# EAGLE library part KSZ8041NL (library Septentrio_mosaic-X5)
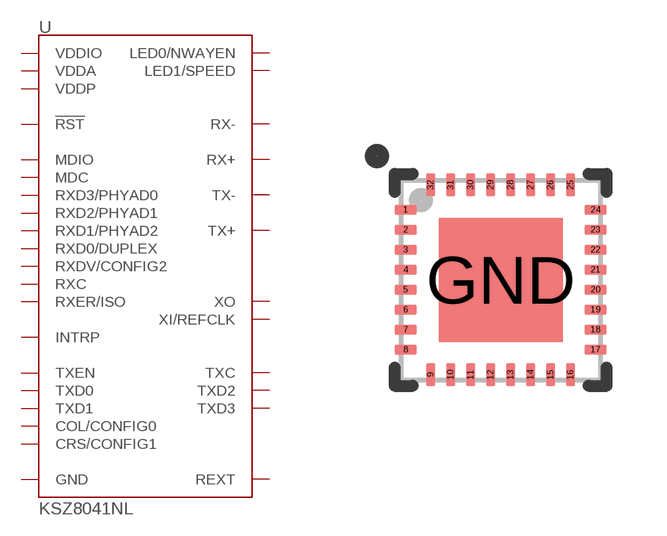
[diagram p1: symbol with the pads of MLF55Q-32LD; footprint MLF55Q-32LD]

Designator prefix -

## KSZ8041NL (PROD_ID: IC-19428; VALUE: KSZ8041NLI)  [MLF55Q-32LD]
1  GND  pwr
2  VDDP
3  VDDA  pwr
4  RX-
5  RX+
6  TX-
7  TX+
8  XO
9  XI/REFCLK
10  REXT
11  MDIO
12  MDC
13  RXD3/PHYAD0
14  RXD2/PHYAD1
15  RXD1/PHYAD2
16  RXD0/DUPLEX
17  VDDIO  pwr
18  RXDV/CONFIG2
19  RXC
20  RXER/ISO
21  INTRP
22  TXC
23  TXEN
24  TXD0
25  TXD1
26  TXD2
27  TXD3
28  COL/CONFIG0
29  CRS/CONFIG1
30  LED0/NWAYEN  out
31  LED1/SPEED  out
32  !RST!
GND  GND  pwr

## Footprint MLF55Q-32LD (pad centres in mm)
smd 0.55 x 0.23: 1 -2.375,1.75; 2 -2.375,1.25; 3 -2.375,0.75; 4 -2.375,0.25; 5 -2.375,-0.25; 6 -2.375,-0.75; 7 -2.375,-1.25; 8 -2.375,-1.75; 17 2.375,-1.75; 18 2.375,-1.25; 19 2.375,-0.75; 20 2.375,-0.25; 21 2.375,0.25; 22 2.375,0.75; 23 2.375,1.25; 24 2.375,1.75
smd 0.23 x 0.55: 9 -1.75,-2.375; 10 -1.25,-2.375; 11 -0.75,-2.375; 12 -0.25,-2.375; 13 0.25,-2.375; 14 0.75,-2.375; 15 1.25,-2.375; 16 1.75,-2.375; 25 1.75,2.375; 26 1.25,2.375; 27 0.75,2.375; 28 0.25,2.375; 29 -0.25,2.375; 30 -0.75,2.375; 31 -1.25,2.375; 32 -1.75,2.375
smd 3.1 x 3.1: GND 0,0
